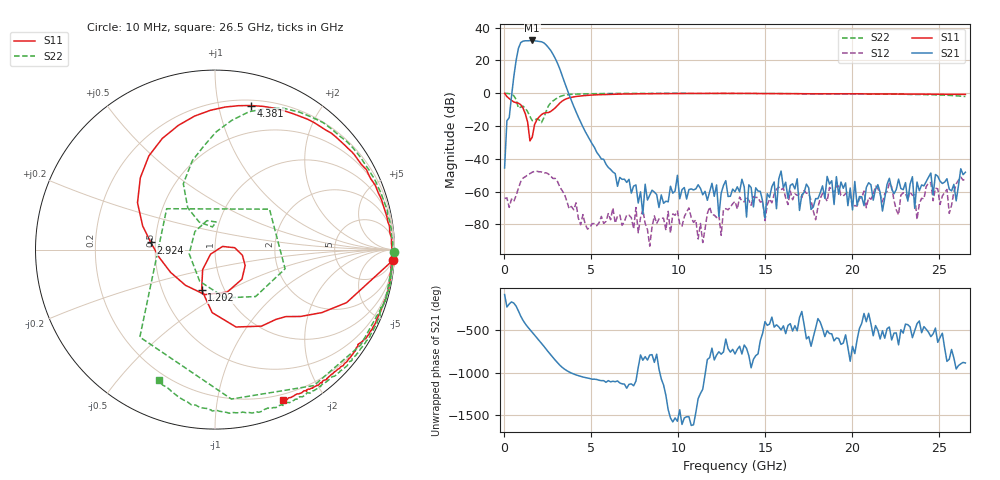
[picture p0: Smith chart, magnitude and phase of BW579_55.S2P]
!Agilent Technologies,N5242A,MY52422126,A.09.90.01
!Agilent N5242A: A.09.90.01
!Date: Thursday, November 19, 2015 09:32:55
!Correction: S11(Full 2 Port(1,2))
!S21(Full 2 Port(1,2))
!S12(Full 2 Port(1,2))
!S22(Full 2 Port(1,2))
!S2P File: Measurements: S11, S21, S12, S22:
# Hz S  dB  R 50
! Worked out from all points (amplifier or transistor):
!   201 points, 10 MHz to 26.5 GHz, reference 50 ohm
!   highest |S21| = 32.2 dB at 1.599 GHz (marker M1)
!   |S21| within 3 dB of that: 873.3 MHz to 2.421 GHz (1.548 GHz wide, 94 % of centre)
!   unconditionally stable (mu >= 1): start of sweep to end of sweep
!   at 4.381 GHz: K = 1074.64, MAG = -2.0 dB, |S12| = -80.2 dB
!   at 13.26 GHz: K = 592.93, MAG = -27.8 dB, |S12| = -66.0 dB
!   at 26.5 GHz: K = 2964.61, MAG = -35.7 dB, |S12| = -52.2 dB
!   S11 on the Smith chart (normalised r, x): 10 MHz: 4, -32; 1.202 GHz: 0.78, -0.37; 2.924 GHz: 0.47, +0.04; 4.381 GHz: 0.25, +1.25; 26.5 GHz: 0.14, -1.54
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1e7  -0.07 -3.5  -45.57 -83.2  -64.22 -87.0  -0.00 -0.8
5.398e8  -5.31 -43.5  10.22 176.1  -65.96 -93.9  -1.54 -83.7
6.7225e8  -5.75 -49.0  20.09 140.4  -62.36 -83.8  -3.84 -130.7
8.047e8  -6.04 -58.7  27.39 83.7  -57.84 -142.9  -9.05 139.8
9.3715e8  -7.00 -74.8  30.90 23.5  -53.92 172.4  -8.45 36.6
1.0696e9  -9.08 -92.6  31.78 -26.5  -51.77 133.7  -7.85 -15.3
1.20205e9  -12.54 -108.4  32.02 -66.9  -50.89 90.5  -9.22 -49.1
1.3345e9  -17.64 -121.7  32.00 -102.9  -49.80 55.8  -11.22 -78.1
1.5994e9  -26.75 22.6  32.21 -167.1  -48.12 -6.0  -16.73 -170.9
1.73185e9  -19.13 5.4  32.04 161.2  -47.67 -35.2  -16.45 138.1
1.99675e9  -14.43 -27.8  31.59 98.4  -47.94 -91.7  -16.25 87.7
2.26165e9  -12.15 -74.1  30.78 31.6  -48.67 -145.8  -15.06 119.8
2.52655e9  -11.76 -129.7  27.90 -36.9  -49.21 160.1  -7.81 115.7
2.9239e9  -8.88 173.6  21.13 -134.2  -51.94 85.8  -3.67 89.5
3.32125e9  -4.77 136.1  10.67 142.4  -59.39 6.0  -1.52 69.6
4.38085e9  -1.64 75.8  -17.59 37.0  -80.20 -28.5  -0.40 36.5
4.5133e9  -1.50 71.4  -20.54 28.9  -74.03 32.9  -0.38 34.2
8.88415e9  -0.22 11.1  -69.68 122.4  -76.69 -147.8  -0.08 -7.3
1.3255e10  -0.10 -14.4  -60.03 -60.2  -65.96 0.4  -0.12 -29.9
1.77583e10  -0.36 -33.8  -69.35 140.0  -71.95 159.3  -0.33 -50.5
2.212915e10  -0.42 -49.6  -51.87 -103.8  -54.95 -155.8  -0.60 -73.0
2.65e10  -0.72 -65.6  -48.19 -166.1  -52.20 -155.9  -2.01 -113.2
